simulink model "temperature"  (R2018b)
settings: Solver=VariableStepAuto  StartTime=0.0  StopTime=200  RelTol=1e-3
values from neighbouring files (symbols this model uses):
  T0 = 18    [initialization.m]

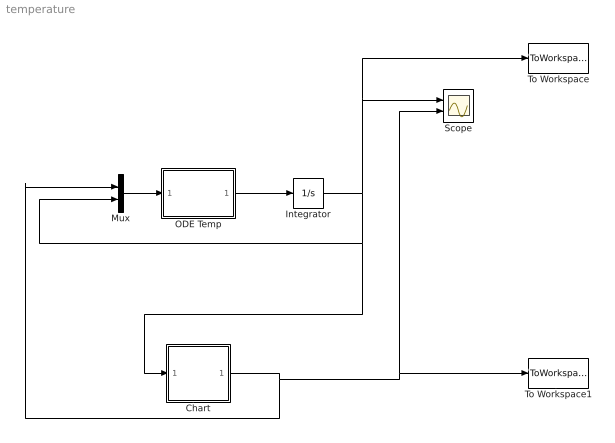
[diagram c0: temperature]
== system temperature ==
  Chart : Stateflow chart  TreatAsAtomicUnit=on
  Integrator : Integrator  InitialCondition=T0
  Mux : Mux  Inputs=2
  ODE Temp : MATLAB Function  TreatAsAtomicUnit=on
  Scope : Scope  NumInputPorts=2
  To Workspace : ToWorkspace  VariableName=T  SampleTime=-1
  To Workspace1 : ToWorkspace  VariableName=h  SampleTime=-1
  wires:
  ODE Temp/1(y) -> Integrator/1
  Integrator/1 -> To Workspace/1, Scope/1, Chart/1(T), Mux/2
  Mux/1 -> ODE Temp/1(u)
  Chart/1(h) -> Mux/1, Scope/2, To Workspace1/1

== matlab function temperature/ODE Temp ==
function y = ODEtemp(u)
% Constant
a = 0.2;  % dec rate
k = 6;

% \var
h = u(1);
T = u(2);

% ODE equation 
dTdt =  -a * T + k * h;

y = [dTdt];

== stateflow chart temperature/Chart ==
  state cooling
    entry:
    h = 0
    T>=18;
  state heating
    entry:
    h = 1
    T<=22;
  (default) -> cooling
  cooling -> heating : [T <= 18]
  heating -> cooling : [T >= 22]
  data: h output; T input
